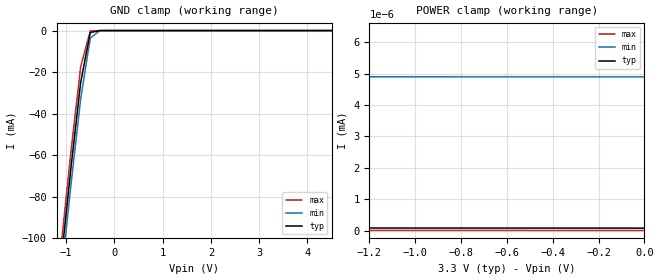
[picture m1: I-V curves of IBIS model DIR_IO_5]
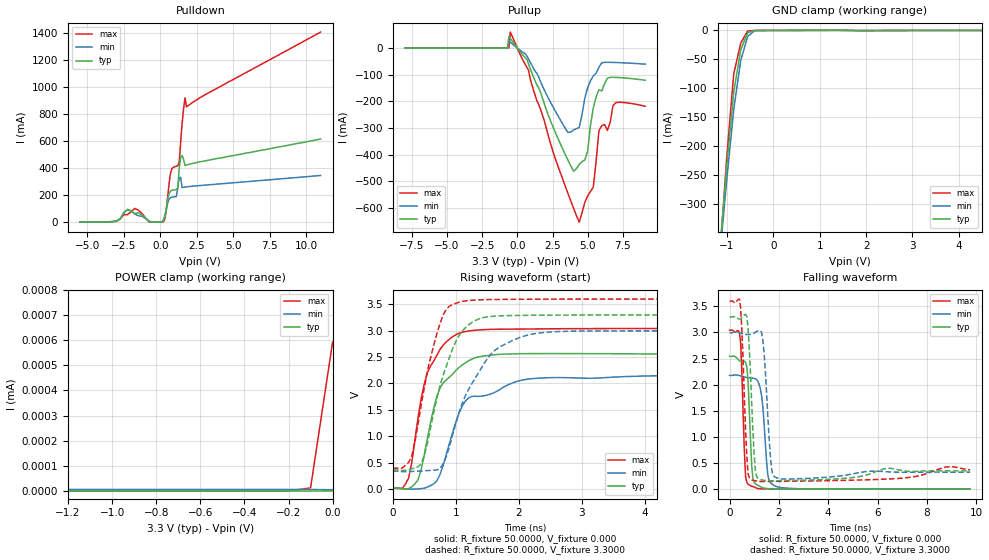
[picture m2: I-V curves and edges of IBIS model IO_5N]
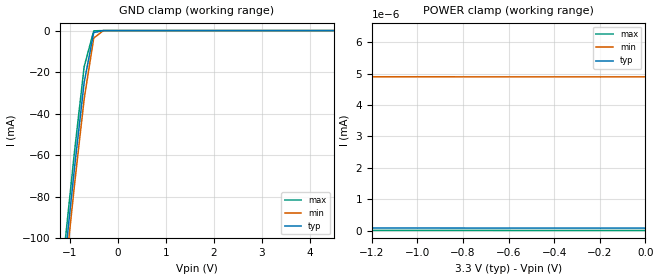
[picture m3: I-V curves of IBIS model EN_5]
| Philips Semiconductors Inc.
| Logic Products Group
| IBIS model of 74LVT245B
| 3.3V Octal transceiver (3-State)
|[Packages]:
|[Package1]: SO 20-pin (D) Package ;
|[Package2]: SSOP 20-Pin Packages ;
|[Package3]: TSSOP 20-pin (PW) Package ;
[IBIS Ver]   3.2
[File Name]   lvt245b.ibs
[File Rev]   1.2
[Date]   22-May-2001
[Source]   File created from simulations by LPG
   Philips Semiconductors Nijmegen
[Notes]   V1.2   Revised model.
[Disclaimer]
   (C) Copyright 2001 Philips Semiconductors
   All rights reserved
   Philips Semiconductors warrants and represents that the IBIS model
   identified herein is owned by Philips Semiconductors (PHILIPS). The
   model provided is not warranted as fully representing all of the
   operating characteristics and specifications of the semiconductor
   products to which the model relates.  Moreover, unless there is a
   signed, written agreement to the contrary, this IBIS model is
   furnished on an "as is" basis without support or warranty of any
   kind, either expressed or implied, regarding the use thereof, and
   PHILIPS specifically disclaims all implied warranties of
   merchantability and fitness of the model for any purpose.
   PHILIPS does not assume any liability arising out of the application
   or use of this IBIS model including infringement of patents and
   copyrights, nor does PHILIPS convey any license under its patents and
   copyrights or the rights of others.
   PHILIPS provides IBIS models as a service to our customers. You and
   your company shall not distribute, convey, sell, or give these models
   to anyone else without receiving prior written permission from
   PHILIPS.
   PHILIPS reserves the right to make changes without notice to these
   IBIS models to improve reliability, function, or design.
   Please be aware that your receipt and subsequent use of the IBIS
   information provided shall serve as acceptance of the terms and
   conditions of this agreement.  If you do not accept these terms,
   you should return or destroy the IBIS models and any other
   accompanying information immediately.
| to specify a consistent format that can be parsed by software, allowing
| simulation vendors to derive models compatible with their own products.
| One goal of this template is to represent the current state of IBIS data,
| while allowing a growth path to more complex models / methods (when deemed
| appropriate).  This would be accomplished by a revision of the base
| template, and possibly the addition of new keywords or categories.
| Another goal of this template is to ensure that it is simple enough for
| semiconductor vendors and customers to use and modify, while ensuring that
| it is rigid enough for simulation vendors to write reliable parsers.
| Finally, this template is meant to contain a complete description of the I/O
| elements on an entire component.  Consequently, several models will need to
| be defined in each file, as well as a table that equates the appropriate
| buffer to the correct pin and signal name.
| Version 3.2 of this electronic template was finalized by an industry-wide
| group of experts representing various companies and interests.  Regular
| "EIA IBIS Open Forum" meetings were held to accomplish this task.
| Commitment to Backward Compatibility.  Version 1.0 is the first valid IBIS
| ASCII file format.  It represents the minimum amount of I/O buffer
| information required to create an accurate IBIS model of common CMOS and
| bipolar I/O structures.  Future revisions of the ASCII file will add items
| considered to be "enhancements" to Version 1.0 to allow accurate modeling
| of new, or other I/O buffer structures.  Consequently, all future revisions
| will be considered supersets of Version 1.0, allowing backward
| compatibility.  In addition, as modeling platforms develop support for
| revisions of the IBIS ASCII template, all previous revisions of the template
| must also be supported.
| Version 1.1 update.  The file "ver1_1.ibs" is conceptually the same as the
| 1.0 version of the IBIS ASCII format (ver1_0.ibs).  However, various
| comments have been added for further clarification.
| Version 2.0 update.  The file "ver2_0.ibs" maintains backward compatibility
| with Versions 1.0 and 1.1.  All new keywords and elements added in Version
| 2.0 are optional.  A complete list of changes to the specification is in the
| IBIS Version 2.0 Release Notes document ("ver2_0.rn").
| Version 2.1 update.  The file "ver2_1.ibs" contains clarification text
| changes, corrections, and two additional waveform parameters beyond
| Version 2.0.
| Version 3.0 update.  The file "ver3_0.ibs" adds a number of new keywords
| and functionality.  A complete list of functions can be found on eda.org
| under /pub/ibis/birds/birddir.txt showing the approved Buffer Issue
| Resolution Documents (BIRDs) that have been approved for Version 3.0.
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[Component]   74LVT245B_1
[Manufacturer]   Philips Semiconductors Inc.
[Package]
|   typ   min   max
R_pkg   5.95E-02   5.36E-02   6.59E-02
L_pkg   4.21E-09   3.07E-09   5.91E-09
C_pkg   0.910E-12  0.758E-12  1.110E-12
[Pin]   signal_name   model_name   R_pin   L_pin   C_pin
   1   DIR   DIR_IO_5 5.75E-02 5.91E-09 1.050E-12
   2   A0   IO_5N 6.25E-02 4.85E-09 1.040E-12
   3   A1   IO_5N 6.59E-02 3.92E-09 0.861E-12
   4   A2   IO_5N 5.79E-02 3.32E-09 0.803E-12
   5   A3   IO_5N 5.36E-02 3.07E-09 0.758E-12
   6   A4   IO_5N 5.36E-02 3.07E-09 0.758E-12
   7   A5   IO_5N 5.79E-02 3.32E-09 0.803E-12
   8   A6   IO_5N 6.59E-02 3.92E-09 0.861E-12
   9   A7   IO_5N 6.25E-02 4.85E-09 1.040E-12
   10   Gnd   GND 5.75E-02 5.91E-09 1.110E-12
   11   B7   IO_5N 5.75E-02 5.91E-09 1.110E-12
   12   B6   IO_5N 6.25E-02 4.85E-09 1.040E-12
   13   B5   IO_5N 6.59E-02 3.92E-09 0.861E-12
   14   B4   IO_5N 5.79E-02 3.32E-09 0.803E-12
   15   B3   IO_5N 5.36E-02 3.07E-09 0.758E-12
   16   B2   IO_5N 5.36E-02 3.07E-09 0.758E-12
   17   B1   IO_5N 5.79E-02 3.32E-09 0.803E-12
   18   B0   IO_5N 6.59E-02 3.92E-09 0.861E-12
   19   OE#   EN_5 6.25E-02 4.85E-09 1.040E-12
   20   Vcc   POWER 5.75E-02 5.91E-09 1.110E-12
|   Info for  SSOP 20-Pin Packages
[Component]   74LVT245B_2
[Manufacturer]   Philips Semiconductors Inc.
[Package]
|   typ   min   max
R_pkg   50.90m   43.00m   62.10m
L_pkg   2.37nH   1.87nH   3.04nH
C_pkg   0.62pF   0.55pF   0.71pF
[Pin]   signal_name   model_name   R_pin   L_pin   C_pin
   1   DIR   DIR_IO_5   47.20m   3.04nH   0.65pF
   2   A0   IO_5N   51.40m   2.60nH   0.70pF
   3   A1   IO_5N   62.10m   2.31nH   0.59pF
   4   A2   IO_5N   50.80m   2.03nH   0.58pF
   5   A3   IO_5N   43.00m   1.87nH   0.56pF
   6   A4   IO_5N   43.00m   1.87nH   0.56pF
   7   A5   IO_5N   50.80m   2.03nH   0.58pF
   8   A6   IO_5N   62.10m   2.31nH   0.59pF
   9   A7   IO_5N   51.40m   2.60nH   0.70pF
   10   Gnd   GND   47.20m   3.04nH   0.69pF
   11   B7   IO_5N   47.20m   3.05nH   0.69pF
   12   B6   IO_5N   51.40m   2.60nH   0.70pF
   13   B5   IO_5N   62.10m   2.32nH   0.59pF
   14   B4   IO_5N   50.80m   2.03nH   0.58pF
   15   B3   IO_5N   43.00m   1.88nH   0.55pF
   16   B2   IO_5N   43.00m   1.87nH   0.55pF
   17   B1   IO_5N   50.80m   2.03nH   0.58pF
   18   B0   IO_5N   62.10m   2.31nH   0.59pF
   19   OE#   EN_5   51.40m   2.60nH   0.71pF
   20   Vcc   POWER   47.50m   3.00nH   0.68pF
|   Info for  TSSOP 20-pin (PW) Package
[Component]   74LVT245B_3
[Manufacturer]   Philips Semiconductors Inc.
[Package]
|   typ   min   max
R_pkg   7.24E-02   6.63E-02   8.34E-02
L_pkg   2.47E-09   2.09E-09   3.18E-09
C_pkg   0.341E-12  0.282E-12  0.420E-12
[Pin]   signal_name   model_name   R_pin   L_pin   C_pin
   1   DIR   DIR_IO_5 6.63E-02 3.18E-09 0.408E-12
   2   A0   IO_5N 6.67E-02 2.55E-09 0.398E-12
   3   A1   IO_5N 8.34E-02 2.35E-09 0.317E-12
   4   A2   IO_5N 7.44E-02 2.16E-09 0.293E-12
   5   A3   IO_5N 7.10E-02 2.09E-09 0.282E-12
   6   A4   IO_5N 7.10E-02 2.09E-09 0.282E-12
   7   A5   IO_5N 7.44E-02 2.16E-09 0.293E-12
   8   A6   IO_5N 8.34E-02 2.35E-09 0.317E-12
   9   A7   IO_5N 6.67E-02 2.55E-09 0.397E-12
   10   Gnd   GND 6.63E-02 3.18E-09 0.420E-12
   11   B7   IO_5N 6.63E-02 3.17E-09 0.420E-12
   12   B6   IO_5N 6.67E-02 2.55E-09 0.397E-12
   13   B5   IO_5N 8.34E-02 2.35E-09 0.317E-12
   14   B4   IO_5N 7.44E-02 2.16E-09 0.293E-12
   15   B3   IO_5N 7.10E-02 2.09E-09 0.282E-12
   16   B2   IO_5N 7.10E-02 2.09E-09 0.282E-12
   17   B1   IO_5N 7.44E-02 2.16E-09 0.293E-12
   18   B0   IO_5N 8.34E-02 2.35E-09 0.317E-12
   19   OE#   EN_5 6.67E-02 2.55E-09 0.398E-12
   20   Vcc   POWER 6.63E-02 3.17E-09 0.420E-12
| Models and submodels in the file (3): DIR_IO_5 (Input), IO_5N (I/O), EN_5 (Input)
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|   Model DIR_IO_5
[Model]   DIR_IO_5
Model_type   Input
Polarity   Non-Inverting
Vinl =   0.8000V
Vinh =   2.0000V
C_comp   2.8pF   1.5pF   4.1pF
[Model Spec]
| Note: The input and output voltage ratings may be exceeded if the input and
|   output current ratings are observed (please refer to the data sheet)
|   Subparameter   typ   min   max
| Thresholds
Vinh   2.0   NA   NA
Vinl   0.8   NA   NA
| Overshoot
S_overshoot_high   4.6   4.6   4.6   | Static overshoot
S_overshoot_low   -0.5   -0.5   -0.5
D_overshoot_high   7.2   7.2   7.2   | Dynamic overshoot
D_overshoot_low   -3.6   -3.6   -3.6
D_overshoot_time   3n   3n   3n
| Timing Thresholds
Vmeas   1.5   1.5   1.5
[Temperature Range]   25.0000   85.0000   -40.0000
| Remark: The curves below are the result of a simulation using the following
| die temperatures:   55.0000   110.0000   0.0000
[Voltage Range]   3.3000V   3.0000V   3.6000V
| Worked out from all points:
|   GND clamp passes 1 mA (typ) near -0.50 V on its own axis
|   POWER clamp passes 1 mA (typ) near -4.81 V on its own axis
|Process Range   nominal   slow   fast
[GND_clamp]
| voltage   I(typ)   I(min)   I(max)
-5.5V     -1.144A    -1.15A     -1.139A
-1.1V     -110.1mA   -118.1mA   -102.6mA
-900mV    -65.97mA   -74.13mA   -58.16mA
-700mV    -25.02mA   -33mA      -17.44mA
-500mV    -923.8uA   -3.598mA   -124.2uA
-300mV    -2.053uA   -27.18uA   -52.17nA
5.5V      92.2pA     4.901nA    16.74pA
[POWER_clamp]
| voltage   I(typ)   I(min)   I(max)
-8V       574.1mA    551.7mA    596.8mA
-4V       2.435uA    8.749nA    150.6uA
-3.9V     75.97nA    5.092nA    56.04uA
-3.8V     2.311nA    4.915nA    4.695uA
-3.7V     161.2pA    4.906nA    78.65nA
-3.6V     98.27pA    4.905nA    1.148nA
-3.5V     96.15pA    4.905nA    37.63pA
0V        85.6pA     4.893nA    11.04pA
|   Model IO_5N
[Model]   IO_5N
Model_type   I/O
Polarity   Non-Inverting
Enable   Active-Low
Vinl =   0.8000V
Vinh =   2.0000V
Vmeas =   1.5000V
Cref =  50.0000pF
Rref =   0.5000k
Vref =  0.000V
C_comp   7.8pF   4.9pF   10.7pF
[Model Spec]
| Note: The input and output voltage ratings may be exceeded if the input and
|   output current ratings are observed (please refer to the data sheet)
|   Subparameter   typ   min   max
| Overshoot
S_overshoot_high   4.6   4.6   4.6   | Static overshoot
S_overshoot_low   -0.5   -0.5   -0.5
D_overshoot_high   7.2   7.2   7.2   | Dynamic overshoot
D_overshoot_low   -3.6   -3.6   -3.6
D_overshoot_time   3n   3n   3n
| Timing Thresholds
Vmeas   1.5   1.5   1.5
[Temperature Range]   25.0000   85.0000   -40.0000
| Remark: The curves below are the result of a simulation using the following
| die temperatures:   55.0000   110.0000   0.0000
[Voltage Range]   3.3000V   3.0000V   3.6000V
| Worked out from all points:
|   slope of the pulldown table from 0 to 0.495 V, typ, clamps not added: 3.18 ohm
|   slope of the pullup table from 0 to 0.495 V, typ, clamps not added: 15.3 ohm
|   GND clamp passes 1 mA (typ) near -0.44 V on its own axis
|   POWER clamp passes 1 mA (typ) near -4.81 V on its own axis
|   rising waveform, R_fixture 50.0000, V_fixture 0.000: 20-80 % time 346ps typ, 434ps min, 340ps max; typ from 0.006 V to 2.54 V
|   rising waveform, R_fixture 50.0000, V_fixture 3.3000: 20-80 % time 406ps typ, 587ps min, 332ps max; typ from 0.355 V to 3.3 V
|   falling waveform, R_fixture 50.0000, V_fixture 0.000: 20-80 % time 139ps typ, 208ps min, 131ps max; typ from 2.54 V to 0.005 V
|   falling waveform, R_fixture 50.0000, V_fixture 3.3000: 20-80 % time 169ps typ, 200ps min, 155ps max; typ from 3.3 V to 0.355 V
|Process Range   nominal   slow   fast
[Pulldown]
| voltage   I(typ)   I(min)   I(max)
-5.5V     360.4uA    300.7uA    389.8uA
-3V       6.319mA    5.021mA    8.899mA
-1.75V    62.63mA    60.4mA     100.5mA
200mV     5.641mA    11.17mA    1.097mA
400mV     88.44mA    88.45mA    72.53mA
700mV     229.3mA    180.6mA    359.3mA
1.2V      253.3mA    249.6mA    416.6mA
1.3V      394.8mA    326.6mA    441mA
1.5V      493.8mA    255.3mA    729.6mA
1.7V      418.9mA    259.2mA    920.9mA
1.8V      422.5mA    260.8mA    854mA
11V       615.4mA    345.1mA    1.409A
[Pullup]
| voltage   I(typ)   I(min)   I(max)
-8V       63.45uA    30.08uA    128uA
-600mV    43.5mA     26.4mA     108.8uA
-500mV    36.16mA    21.96mA    60.11mA
3.6V      -420.9mA   -316.4mA   -545.7mA
4.4V      -436.3mA   -297.8mA   -653.6mA
5V        -386.4mA   -147.9mA   -554.6mA
5.2V      -290mA     -122.7mA   -538.3mA
5.4V      -224.2mA   -104.6mA   -522.2mA
5.8V      -156.2mA   -71.4mA    -309.8mA
6.4V      -112.8mA   -53.29mA   -308.7mA
6.8V      -109.7mA   -53.75mA   -215.8mA
9.1V      -120.8mA   -60.39mA   -218.4mA
[GND_clamp]
| voltage   I(typ)   I(min)   I(max)
-5.5V     -10.31A    -8.927A    -8.632A
-1.15V    -378.3mA   -389.3mA   -391.9mA
-1V       -234.7mA   -258mA     -218.2mA
-850mV    -106.6mA   -136.5mA   -74.91mA
-700mV    -33.54mA   -52.14mA   -21.93mA
-550mV    -3.842mA   -10.31mA   -881.5uA
-400mV    -114.3uA   -411.2uA   -64.81uA
-250mV    -39.36uA   -40.9uA    -38.37uA
5.5V      235.5pA    5.957nA    743.9pA
[POWER_clamp]
| voltage   I(typ)   I(min)   I(max)
-8V       629.3mA    604.4mA    654.8mA
-4.2V     114.9uA    1.588uA    371.5uA
-4.1V     33.94uA    85.38nA    258.6uA
-4V       2.438uA    9.844nA    150.8uA
-3.9V     76.24nA    6.18nA     56.1uA
-3.8V     2.499nA    6.001nA    4.703uA
-3.7V     344.5pA    5.989nA    81.12nA
-3.6V     278.4pA    5.986nA    3.369nA
-200mV    169.6pA    5.889nA    225.9pA
-100mV    180.8pA    5.785nA    12.31nA
0V        192.7pA    5.047nA    593nA
[Ramp]
| variable   typ   min   max
dV/dt_r  1.523E+00/346.190E-12  1.301E+00/433.312E-12  1.822E+00/340.417E-12
dV/dt_f  1.767E+00/168.557E-12  1.602E+00/200.034E-12  1.936E+00/154.959E-12
R_load = 50.0000
[Rising Waveform]
R_fixture = 50.0000
V_fixture = 0.000
V_fixture_min = 0.000
V_fixture_max = 0.000
| time   V(typ)   V(min)   V(max)
0s        6.399mV    6.207mV    5.977mV
150ps     -2.529mV   4.517mV    8.457mV
250ps     3.87mV     -5.467mV   200.2mV
400ps     169.8mV    -189.7uV   1.343V
550ps     963mV      33.69mV    2.205V
700ps     1.754V     154.5mV    2.533V
1.1ns     2.347V     1.567V     2.971V
1.25ns    2.458V     1.752V     3.002V
2.35ns    2.566V     2.102V     3.034V
9.75ns    2.544V     2.175V     3.043V
[Rising Waveform]
R_fixture = 50.0000
V_fixture = 3.3000
V_fixture_min = 3.0000
V_fixture_max = 3.6000
| time   V(typ)   V(min)   V(max)
0s        354.9mV    330.7mV    389.8mV
300ps     378.7mV    330.5mV    617.3mV
450ps     474.1mV    337.1mV    1.579V
600ps     1.156V     352.1mV    2.488V
800ps     2.158V     471.8mV    3.301V
1.05ns    2.903V     1.443V     3.54V
1.2ns     3.107V     1.879V     3.572V
1.6ns     3.275V     2.609V     3.592V
2.3ns     3.294V     2.952V     3.597V
9.75ns    3.3V       2.999V     3.6V
[Falling Waveform]
R_fixture = 50.0000
V_fixture = 0.000
V_fixture_min = 0.000
V_fixture_max = 0.000
| time   V(typ)   V(min)   V(max)
0s        2.545V     2.182V     3.044V
400ps     2.461V     2.177V     3.004V
450ps     2.45V      2.169V     2.799V
650ps     2.425V     2.144V     244.6mV
800ps     1.53V      2.133V     84.59mV
950ps     186.2mV    2.127V     54.02mV
1.25ns    54.79mV    1.919V     12.57mV
1.55ns    15.89mV    277.6mV    9.047mV
1.85ns    9.665mV    64.85mV    8.15mV
9.75ns    5.38mV     5.147mV    5.426mV
[Falling Waveform]
R_fixture = 50.0000
V_fixture = 3.3000
V_fixture_min = 3.0000
V_fixture_max = 3.6000
| time   V(typ)   V(min)   V(max)
0s        3.3V       3V         3.6V
450ps     3.264V     2.987V     3.466V
700ps     3.307V     2.961V     637mV
850ps     2.206V     2.964V     198.9mV
950ps     1.083V     2.979V     176.9mV
1.05ns    345.2mV    3.005V     166.2mV
1.35ns    177.9mV    2.853V     152mV
1.65ns    164.6mV    664.4mV    152.7mV
1.85ns    165.4mV    234.1mV    153.6mV
9.75ns    354.8mV    330.5mV    373.2mV
|   Model EN_5
[Model]   EN_5
Model_type   Input
Polarity   Non-Inverting
Vinl =   0.8000V
Vinh =   2.0000V
C_comp   2.6pF   1.0pF   4.1pF
[Model Spec]
| Note: The input and output voltage ratings may be exceeded if the input and
|   output current ratings are observed (please refer to the data sheet)
|   Subparameter   typ   min   max
| Thresholds
Vinh   2.0   NA   NA
Vinl   0.8   NA   NA
| Overshoot
S_overshoot_high   4.6   4.6   4.6   | Static overshoot
S_overshoot_low   -0.5   -0.5   -0.5
D_overshoot_high   7.2   7.2   7.2   | Dynamic overshoot
D_overshoot_low   -3.6   -3.6   -3.6
D_overshoot_time   3n   3n   3n
| Timing Thresholds
Vmeas   1.5   1.5   1.5
[Temperature Range]   25.0000   85.0000   -40.0000
| Remark: The curves below are the result of a simulation using the following
| die temperatures:   55.0000   110.0000   0.0000
[Voltage Range]   3.3000V   3.0000V   3.6000V
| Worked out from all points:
|   GND clamp passes 1 mA (typ) near -0.50 V on its own axis
|   POWER clamp passes 1 mA (typ) near -4.81 V on its own axis
|Process Range   nominal   slow   fast
[GND_clamp]
| voltage   I(typ)   I(min)   I(max)
-5.5V     -1.144A    -1.15A     -1.139A
-1.1V     -110.1mA   -118.1mA   -102.6mA
-900mV    -65.97mA   -74.13mA   -58.16mA
-700mV    -25.02mA   -33mA      -17.44mA
-500mV    -923.8uA   -3.598mA   -124.2uA
-300mV    -2.053uA   -27.18uA   -52.17nA
5.5V      92.2pA     4.901nA    16.74pA
[POWER_clamp]
| voltage   I(typ)   I(min)   I(max)
-8V       574.1mA    551.7mA    596.8mA
-4V       2.435uA    8.749nA    150.6uA
-3.9V     75.97nA    5.092nA    56.04uA
-3.8V     2.311nA    4.915nA    4.695uA
-3.7V     161.2pA    4.906nA    78.65nA
-3.6V     98.27pA    4.905nA    1.148nA
-3.5V     96.15pA    4.905nA    37.63pA
0V        85.6pA     4.893nA    11.04pA
